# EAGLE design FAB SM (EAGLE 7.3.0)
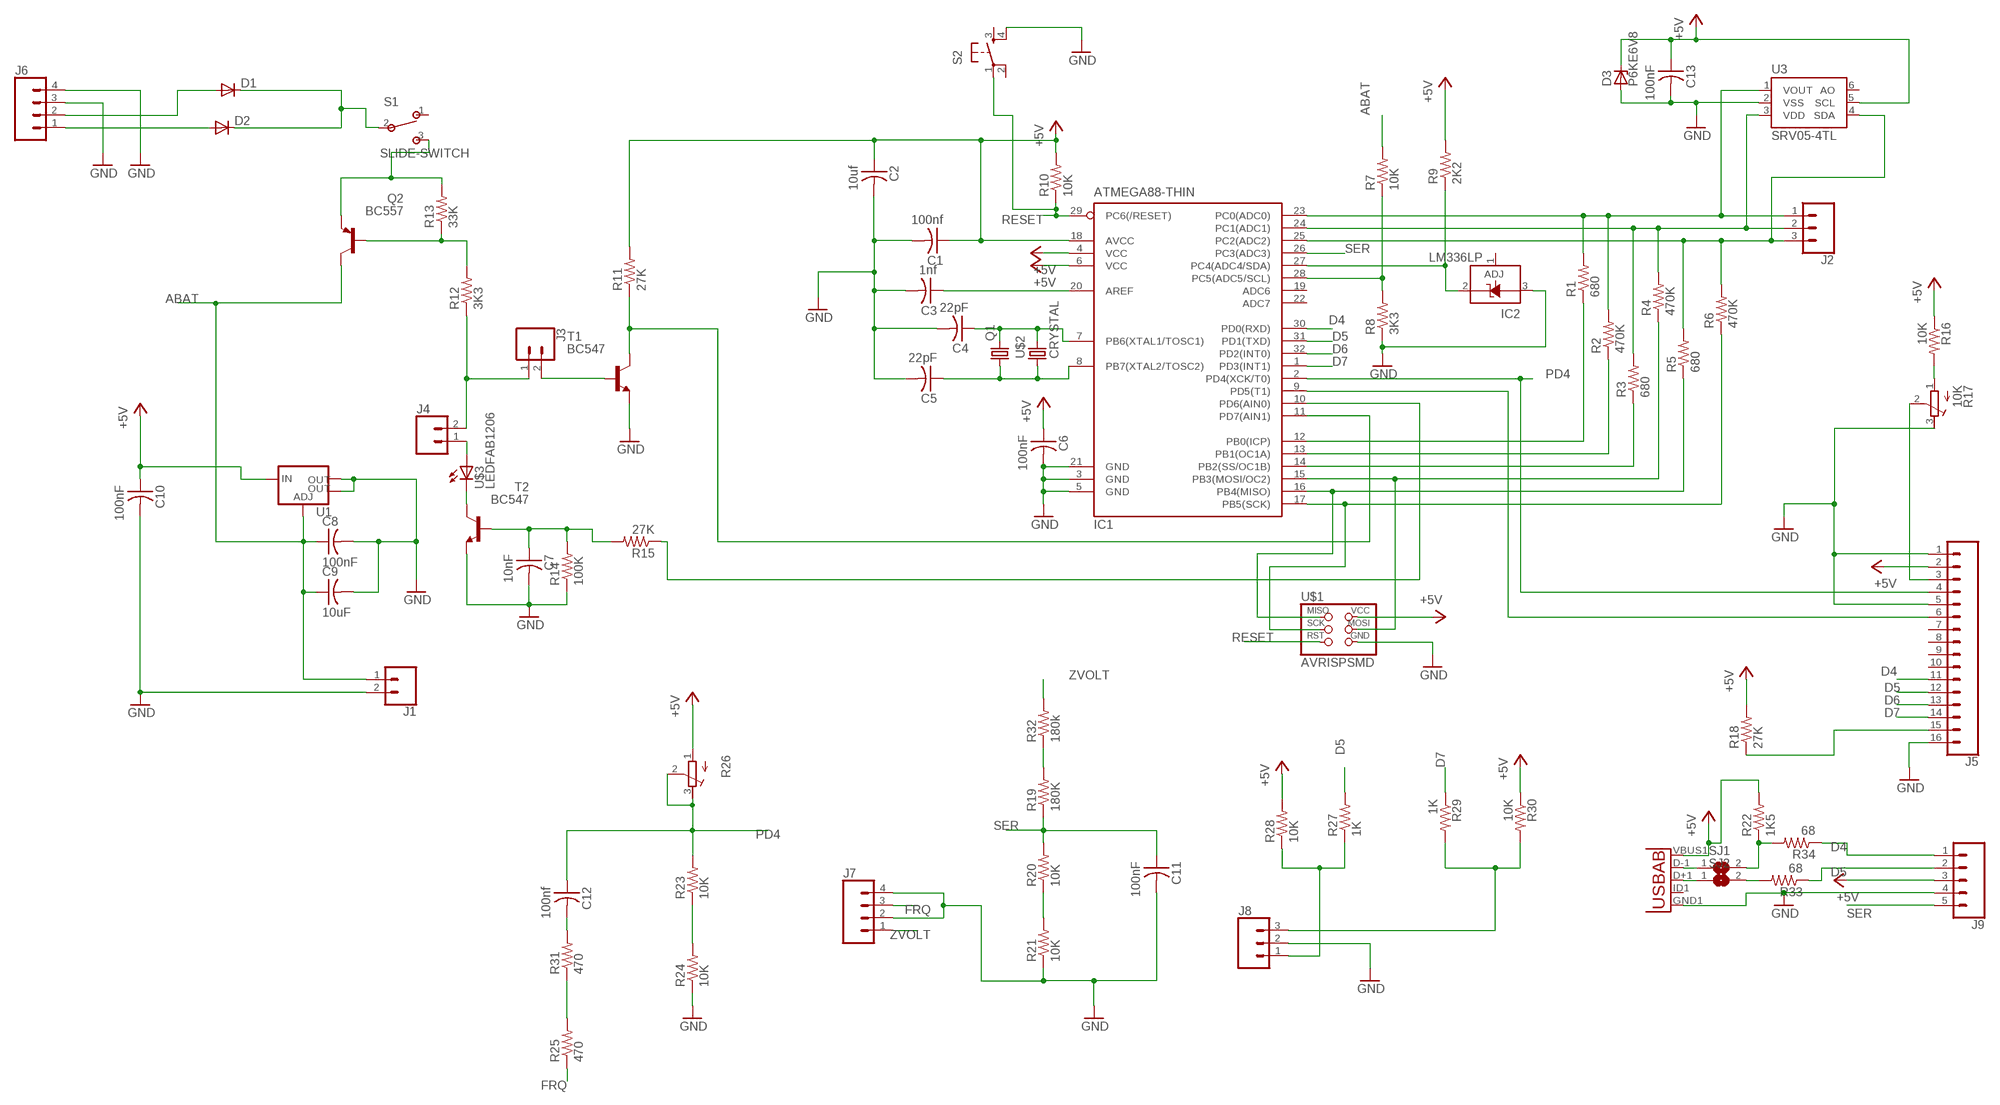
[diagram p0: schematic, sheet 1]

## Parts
C1  100nf  CAP-US1206FAB  [C1206FAB]
C2  10uf  CAP-US1206FAB  [C1206FAB]
C3  1nf  CAP-US1206FAB  [C1206FAB]
C4  22pF  CAP-US1206FAB  [C1206FAB]
C5  22pF  CAP-US1206FAB  [C1206FAB]
C6  100nF  CAP-US1206FAB  [C1206FAB]
C7  10nF  CAP-US1206FAB  [C1206FAB]
C8  100nF  CAP-US1206FAB  [C1206FAB]
C9  10uF  CAP-US1206FAB  [C1206FAB]
C10  100nF  CAP-US1206FAB  [C1206FAB]
C11  100nF  CAP-US1206FAB  [C1206FAB]
C12  100nf  CAP-US1206FAB  [C1206FAB]
C13  100nF  CAP-US1206FAB  [C1206FAB]
D1  DIODESOD123  [SOD123]
D2  DIODESOD123  [SOD123]
D3  P6KE6V8  1N4728  [DO41Z10]
IC1  ATMEGA88-THIN  [TQFP32-08THIN]
IC2  LM336LP  [TO92]
J1  CONN_02PTH3  [1X02_LONGPADS]
J2  CONN_03LOCK_LONGPADS  [1X03_LOCK_LONGPADS]
J3  CONN_02PTH3  [1X02_LONGPADS]
J4  CONN_02PTH3  [1X02_LONGPADS]
J5  CONN_16LONGPADS  [1X16_LONGPADS]
J6  CONN_04LOCK_LONGPADS  [1X04_LOCK_LONGPADS]
J7  CONN_04LOCK_LONGPADS  [1X04_LOCK_LONGPADS]
J8  CONN_03LOCK_LONGPADS  [1X03_LOCK_LONGPADS]
J9  CONN_05LOCK_LONGPADS  [1X05_LOCK_LONGPADS]
Q1  CRYSTALHC49S  [HC49/S]
Q2  BC557  [TO92]
R1  680  RES-US1206FAB  [R1206FAB]
R2  470K  RES-US1206FAB  [R1206FAB]
R3  680  RES-US1206FAB  [R1206FAB]
R4  470K  RES-US1206FAB  [R1206FAB]
R5  680  RES-US1206FAB  [R1206FAB]
R6  470K  RES-US1206FAB  [R1206FAB]
R7  10K  RES-US1206FAB  [R1206FAB]
R8  3K3  RES-US1206FAB  [R1206FAB]
R9  2K2  RES-US1206FAB  [R1206FAB]
R10  10K  RES-US1206FAB  [R1206FAB]
R11  27K  RES-US1206FAB  [R1206FAB]
R12  3K3  RES-US1206FAB  [R1206FAB]
R13  33K  RES-US1206FAB  [R1206FAB]
R14  100K  RES-US1206FAB  [R1206FAB]
R15  27K  RES-US1206FAB  [R1206FAB]
R16  10K  RES-US1206FAB  [R1206FAB]
R17  10K  R-TRIMM64Z  [RTRIM64Z]
R18  27K  RES-US1206FAB  [R1206FAB]
R19  180K  RES-US1206FAB  [R1206FAB]
R20  10K  RES-US1206FAB  [R1206FAB]
R21  10K  RES-US1206FAB  [R1206FAB]
R22  1K5  R-US_0204/7  [0204/7]
R23  10K  RES-US1206FAB  [R1206FAB]
R24  10K  RES-US1206FAB  [R1206FAB]
R25  470  RES-US1206FAB  [R1206FAB]
R26  R-TRIMM64Z  [RTRIM64Z]
R27  1K  RES-US1206FAB  [R1206FAB]
R28  10K  RES-US1206FAB  [R1206FAB]
R29  1K  RES-US1206FAB  [R1206FAB]
R30  10K  RES-US1206FAB  [R1206FAB]
R31  470  R-US_0204/7  [0204/7]
R32  180k  R-US_0204/7  [0204/7]
R33  68  R-US_0204/7  [0204/7]
R34  68  R-US_0204/7  [0204/7]
S1  SLIDE-SWITCH  [AYZ0102AGRLC]
S2  6MM_SWITCH6MM_SWITCH  [6MM_SWITCH]
SJ1  SJ  [SJ]
SJ2  SJ  [SJ]
T1  BC547  [TO92]
T2  BC547  [TO92]
U1  V_REG_LM1117SOT223  [SOT223]
U2  USB""  [USB-MICRO-SMD]
U3  SRV05-4TL  MCP4725SOT-23  [SOT23-6]
U$1  AVRISPSMD  [2X03SMD]
U$2  CRYSTAL  [2-SMD-5X3MM]
U$3  LEDFAB1206  [LED1206FAB]

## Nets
+5V: C1.1 C2.1 C6.1 C10.1 C13.1 D3.C IC1.4(VCC) IC1.6(VCC) IC1.18(AVCC) J5.2 J9.3 R9.2 R10.2 R11.2 R16.1 R18.2 R22.2 R26.1(A) R28.2 R30.1 U1.3(IN) U2.VBUS1(VBUS) U3.5(SCL) U$1.2(VCC)
ABAT: C8.1 C9.1 J1.1 Q2.3(C) R7.2 U1.1(ADJ)
D4: IC1.30(PD0(RXD)) J5.11 J9.1 R34.1
D5: IC1.31(PD1(TXD)) J5.12 J9.2 R27.2 R33.1
D6: IC1.32(PD2(INT0)) J5.13
D7: IC1.1(PD3(INT1)) J5.14 R29.1
FRQ: J7.3 R25.1
GND: C1.2 C2.2 C3.2 C4.2 C5.2 C6.2 C7.2 C8.2 C9.2 C10.2 C11.2 C13.2 D3.A IC1.3(GND) IC1.5(GND) IC1.21(GND) IC2.3(A) J1.2 J5.1 J5.5 J5.16 J6.3 J6.4 J7.2 J7.4 J8.2 J9.4 R8.1 R14.1 R17.3(E) R21.1 R24.1 S2.4(S1) T1.1(E) T2.1(E) U1.2(OUT) U1.4(OUT) U2.GND1(GND) U3.2(VSS) U$1.6(GND)
N$1: IC1.23(PC0(ADC0)) J2.1 R1.2 R2.2 U3.1(VOUT)
N$2: IC1.12(PB0(ICP)) R1.1
N$3: IC1.13(PB1(OC1A)) R2.1
N$4: IC1.14(PB2(SS/OC1B)) R3.1
N$5: IC1.15(PB3(MOSI/OC2)) R4.1 U$1.4(MOSI)
N$6: IC1.16(PB4(MISO)) R5.1 U$1.1(MISO)
N$7: IC1.17(PB5(SCK)) R6.1 U$1.3(SCK)
N$8: IC1.24(PC1(ADC1)) J2.2 R3.2 R4.2 U3.3(VDD)
N$9: IC1.25(PC2(ADC2)) J2.3 R5.2 R6.2 U3.4(SDA)
N$10: IC1.28(PC5(ADC5/SCL)) R7.1 R8.2
N$11: IC1.27(PC4(ADC4/SDA)) IC2.2(C) R9.1
N$12: C3.1 IC1.20(AREF)
N$13: IC1.11(PD7(AIN1)) R11.1 T1.3(C)
N$14: C4.1 IC1.7(PB6(XTAL1/TOSC1)) Q1.2 U$2.P$2
N$15: C5.1 IC1.8(PB7(XTAL2/TOSC2)) Q1.1 U$2.P$1
N$17: J3.2 T1.2(B)
N$18: J3.1 J4.2 R12.1
N$19: Q2.2(B) R12.2 R13.1
N$20: D1.CATHODE(C) D2.CATHODE(C) S1.2
N$21: J4.1 U$3.1(A)
N$22: T2.3(C) U$3.2(C)
N$24: C7.1 R14.2 R15.2 T2.2(B)
N$25: R16.2 R17.1(A)
N$26: IC1.10(PD6(AIN0)) R15.1
N$27: R20.1 R21.2
N$28: J5.3 R17.2(S)
N$29: J8.1 R27.1 R28.1
N$30: J5.15 R18.1
N$31: IC1.9(PD5(T1)) J5.6
N$32: D1.ANODE(A) J6.2
N$33: D2.ANODE(A) J6.1
N$34: R19.2 R32.1
N$35: R23.1 R24.2
N$36: Q2.1(E) R13.2 S1.3
N$37: J8.3 R29.2 R30.2
N$38: R25.2 R31.1
N$39: C12.2 R31.2
N$40: SJ1.1 U2.D-1(D-)
N$42: SJ2.1 U2.D+1(D+)
N$43: R33.2 SJ2.2
N$45: R22.1 R34.2 SJ1.2
PD4: C12.1 IC1.2(PD4(XCK/T0)) J5.4 R23.2 R26.2(S) R26.3(E)
RESET: IC1.29(PC6(/RESET)) R10.1 S2.1(P) U$1.5(RST)
SER: C11.1 IC1.26(PC3(ADC3)) J9.5 R19.1 R20.2
ZVOLT: J7.1 R32.2
Unconnected: IC1.19(ADC6) IC1.22(ADC7) IC2.1(ADJ) J5.7 J5.8 J5.9 J5.10 S1.1 S2.2(P1) S2.3(S) U2.ID1(USBID) U3.6(AO)

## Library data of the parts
C1-C13 = fab:CAP-US
D1 D2 = fab:DIODE: DIODE
D3 = diode:1N4728: Z DIODE
IC1 = fab:ATMEGA88-THIN
IC2 = linear:LM336: 2.5-V INTEGRATED REFERENCE CIRCUITS LM236 Source: http://focus.ti.com/lit/ds/symlink/lm336-2.5.pdf
J1 J3 J4 = SparkFun-Connectors:CONN_02: Multi connection point. Often used as Generic Header-pin footprint for 0.1 inch spaced/style header connections
J2 J8 = SparkFun-Connectors:CONN_03: Multi connection point. Often used as Generic Header-pin footprint for 0.1 inch spaced/style header connections On any of the 0.1 inch spaced packages, you can populate with these: Break Away Headers - Straight (PRT-00116) Break Away Male Headers - Right Angle (PRT-00553) Female Headers (PRT-00115)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
J5 = SparkFun-Connectors:CONN_16: Multi connection point. Often used as Generic Header-pin footprint for 0.1 inch spaced/style header connections On any of the 0.1 inch spaced packages, you can populate with these: Break Away Headers - Straight (PRT-00116) Break Away Male Headers - Right Angle (PRT-00553) Female Headers (PRT-00115)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
J6 J7 = SparkFun-Connectors:CONN_04: Multi connection point. Often used as Generic Header-pin footprint for 0.1 inch spaced/style header connections On any of the 0.1 inch spaced packages, you can populate with these: Break Away Headers - Straight (PRT-00116) Break Away Male Headers - Right Angle (PRT-00553) Female Headers (PRT-00115)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; PROD_ID: CONN-09696
J9 = SparkFun-Connectors:CONN_05: Multi connection point. Often used as Generic Header-pin footprint for 0.1 inch spaced/style header connections On any of the 0.1 inch spaced packages, you can populate with these: Break Away Headers - Straight (PRT-00116) Break Away Male Headers - Right Angle (PRT-00553) Female Headers (PRT-00115)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
Q1 = crystal:CRYSTAL: CRYSTAL; OC_FARNELL: 1667008; OC_NEWARK: unknown
Q2 = transistor-pnp:BC557: PNP Transistor
R1-R16 R18-R21 R23-R25 R27-R30 = fab:RES-US: Resistor (US Symbol)
R17 R26 = resistor:R-TRIMM: Trimm resistor
R22 R31-R34 = resistor:R-US_: RESISTOR, American symbol
S1 = fab:SLIDE-SWITCH: SMD slide-switch AYZ0102AGRLC as found in the fablab inventory. Includes the mounting holes. Made by Zaerc.
S2 = fab:6MM_SWITCH: OMRON SWITCH
SJ1 SJ2 = jumper:SJ: SMD solder JUMPER
T1 T2 = transistor:BC547: NPN TRANSISTOR
U1 = fab:V_REG_LM1117: Voltage Regulator LM1117 Standard adjustable voltage regulator but in SMD form. Spark Fun Electronics SKU : COM-00595; PROD_ID: VREG-08170
U2 = MicroUSB:USB: This is a USB AB connector that is compatible with USB OTG. i.e. this connector can serve as a host or device
U3 = SparkFun-IC-Conversion:MCP4725: MCP4725 DAC Microchip 12-bit I2C DAC, SOT23-6 Datasheet SparkFun Products SparkFun I2C DAC Breakout - MCP4725 (BOB-12918); PROD_ID: IC-08886; VALUE: MCP4725
U$1 = fab:AVRISP
U$2 = fab:CRYSTAL
U$3 = fab:LED: LED

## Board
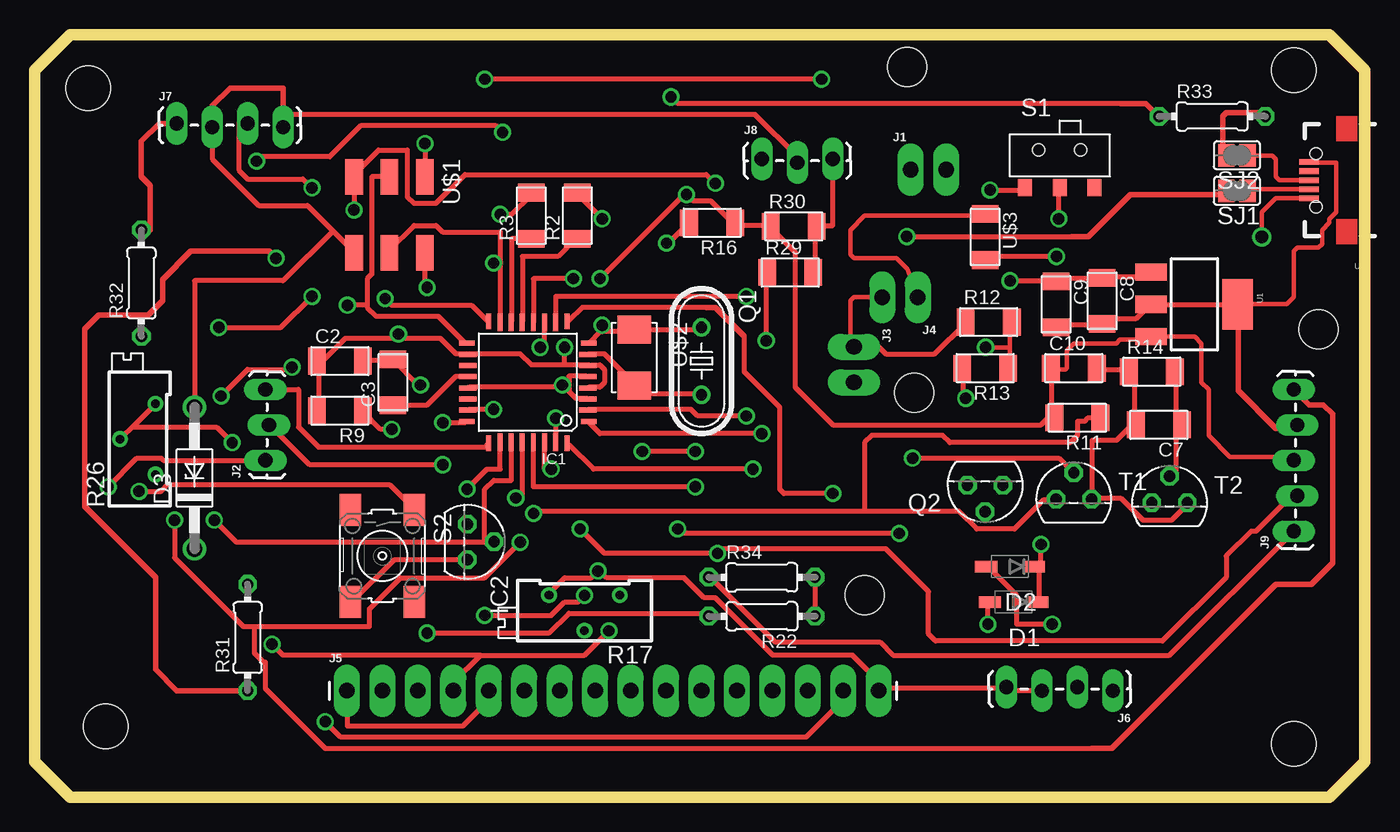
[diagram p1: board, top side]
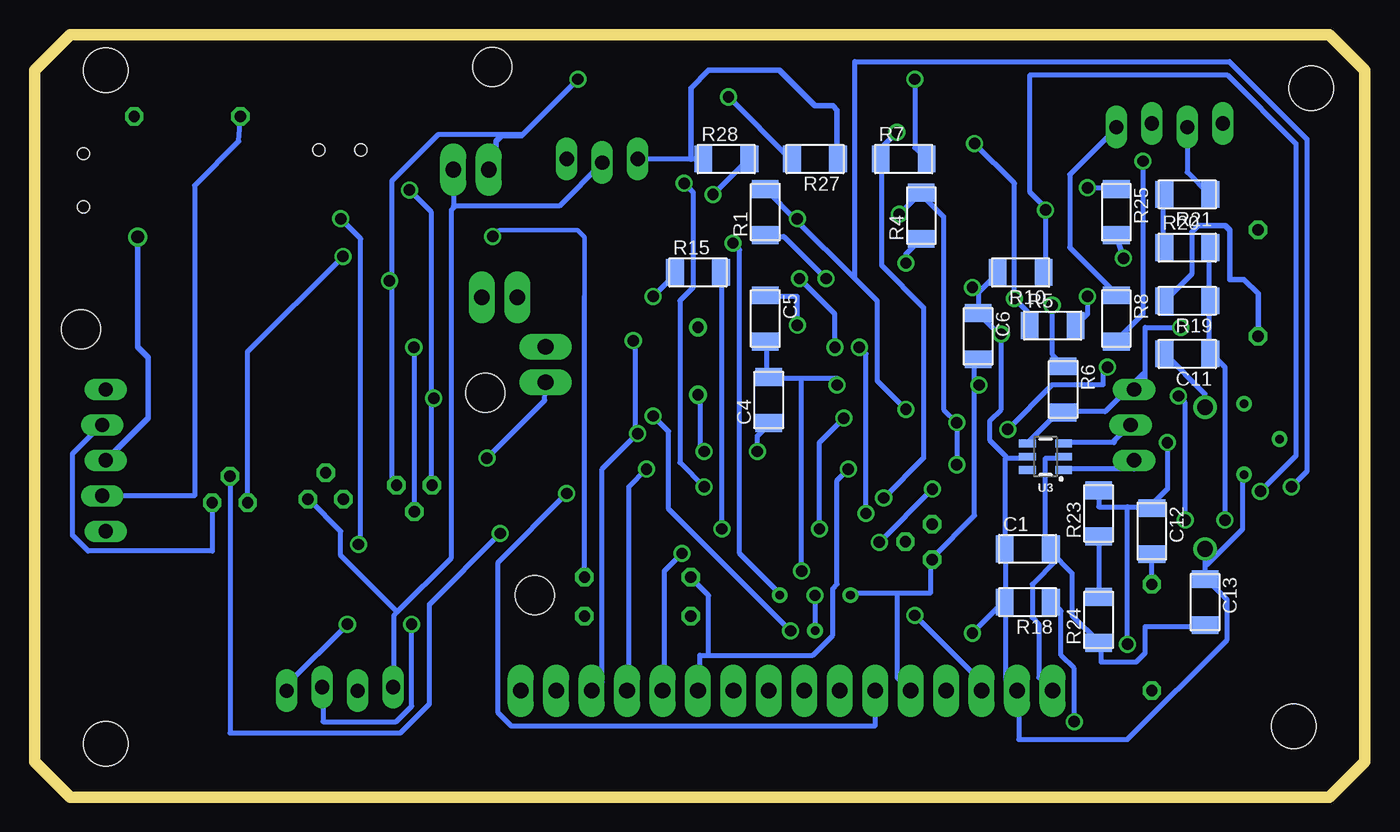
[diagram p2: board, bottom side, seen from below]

Size 95.25 x 54.61 mm. Coordinates in mm from the lower left corner, seen from the top.
Outline: 0,2.54 0,52.07 2.54,54.61 92.71,54.61 95.25,52.07 95.25,2.54 92.71,0 2.54,0 0,2.54
Copper layers (1*16): Top 0.035mm / dielectric 1.5mm / Bottom 0.035mm
Design rules "default *": minimum track width 14mil, minimum drill 32mil, track to track 14mil, track to pad 15mil, pad to pad 16mil, via to via 18mil, smd to smd 14mil, copper to edge 40mil, drill to drill 18mil, minimum pad ring 10mil, minimum via ring 8mil, stop-mask expansion 4mil, vias tented up to drill 0mil, thermal gap 10mil
Holes 3.2 mm at 5.08,5.08 90.17,3.81 90.17,52.07 3.81,50.8
Holes 2.8 mm at 59.44,14.48 62.99,28.96 62.48,52.32 91.95,33.53

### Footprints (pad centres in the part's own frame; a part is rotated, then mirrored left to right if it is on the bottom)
C1206FAB = smd 1.27 x 1.905: 1 -1.651,0; 2 1.651,0
SOD123 = smd 1.6 x 0.8: ANODE 1.7,0; CATHODE -1.7,0
DO41Z10 = drill 1.118: A 5.08,0; C -5.08,0
TQFP32-08THIN = smd 1.118 x 0.356: 1 -4.369,2.8; 8 -4.369,-2.8; 17 4.369,-2.8; 24 4.369,2.8 | smd 1.27 x 0.356: 2 -4.293,2; 3 -4.293,1.2; 4 -4.293,0.4; 5 -4.293,-0.4; 6 -4.293,-1.2; 7 -4.293,-2; 18 4.293,-2; 19 4.293,-1.2; 20 4.293,-0.4; 21 4.293,0.4; 22 4.293,1.2; 23 4.293,2 | smd 0.356 x 1.118: 9 -2.8,-4.369; 16 2.8,-4.369; 25 2.8,4.369; 32 -2.8,4.369 | smd 0.356 x 1.27: 10 -2,-4.293; 14 1.2,-4.293; 15 2,-4.293; 26 2,4.293; 27 1.2,4.293; 31 -2,4.293 | smd 0.35 x 1.27: 11 -1.2,-4.293; 12 -0.4,-4.293; 13 0.4,-4.293; 28 0.4,4.293; 29 -0.4,4.293; 30 -1.2,4.293
TO92 = drill 0.813 octagon: 1 -1.27,0; 2 0,1.905; 3 1.27,0
1X02_LONGPADS = drill 1.118 pad 1.88 long: 1 0,0; 2 2.54,0
1X03_LOCK_LONGPADS = drill 1.016 long: 1 0,0; 2 2.54,-0.254; 3 5.08,0
1X16_LONGPADS = drill 1.118 pad 1.88 long: 1 0,0; 2 2.54,0; 3 5.08,0; 4 7.62,0; 5 10.16,0; 6 12.7,0; 7 15.24,0; 8 17.78,0; 9 20.32,0; 10 22.86,0; 11 25.4,0; 12 27.94,0; 13 30.48,0; 14 33.02,0; 15 35.56,0; 16 38.1,0
1X04_LOCK_LONGPADS = drill 1.016 long: 1 0,0; 2 2.54,-0.254; 3 5.08,0; 4 7.62,-0.254
1X05_LOCK_LONGPADS = drill 1.016 long: 1 0,0; 2 2.54,-0.254; 3 5.08,0; 4 7.62,-0.254; 5 10.16,0
HC49/S = drill 0.813: 1 -2.413,0; 2 2.413,0
TO92' = drill 0.813 octagon: 1 1.27,0; 2 0,1.905; 3 -1.27,0
R1206FAB = smd 1.27 x 1.905: 1 -1.651,0; 2 1.651,0
RTRIM64Z = drill 0.61: 1 0,-2.54; 2 -2.54,0; 3 0,2.54
0204/7 = drill 0.813 octagon: 1 -3.81,0; 2 3.81,0
AYZ0102AGRLC = smd 1 x 1.2: 1 2.5,-2.3; 2 0,-2.3; 3 -2.5,-2.3 | hole 0.85: -1.5,0.4; 1.5,0.4
6MM_SWITCH = smd 2.286 x 1.524: 1 -3.302,2.286; 2 3.302,2.286; 3 -3.302,-2.286; 4 3.302,-2.286
SJ = smd 1.168 x 1.6: 1 -0.762,0; 2 0.762,0
SOT223 = smd 1.219 x 2.235: 1 -2.311,-3.099; 2 0,-3.099; 3 2.311,-3.099 | smd 3.6 x 2.2: 4 0,3.099
USB-MICRO-SMD = smd 1.4 x 0.4: D+1 2.7,0; D-1 2.7,0.65; GND1 2.7,-1.3; ID1 2.7,-0.65; VBUS1 2.7,1.3 | hole 0.85: 2.2,1.9; 2.2,-1.9
SOT23-6 = smd 0.55 x 1.2: 1 0.95,1.3; 2 0,1.3; 3 -0.95,1.3; 4 -0.95,-1.3; 5 0,-1.3; 6 0.95,-1.3
2X03SMD = smd 2.54 x 1.27: 1 -2.54,2.54; 2 2.92,2.54; 3 -2.54,0; 4 2.92,0; 5 -2.54,-2.54; 6 2.92,-2.54
2-SMD-5X3MM = smd 2 x 2.4: P$1 -2,0; P$2 2,0
LED1206FAB = smd 1.27 x 1.905: 1 -1.651,0; 2 1.651,0

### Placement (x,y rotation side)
C1  24.13,17.78 0 bottom
C2  21.84,31.24 0 top
C3  25.65,29.72 90 top
C4  42.67,28.45 90 bottom
C5  42.93,34.29 270 bottom
C6  27.69,33.02 270 bottom
C7  80.52,26.67 180 top
C8  76.45,35.56 270 top
C9  73.15,35.31 270 top
C10  74.42,30.73 0 top
C11  12.7,31.75 180 bottom
C12  15.24,19.05 270 bottom
C13  11.43,13.97 270 bottom
D1  70.1,13.97 180 top
D2  69.85,16.51 180 top
D3  11.43,22.86 90 top
IC1  35.31,29.72 180 top
IC2  30.99,18.29 270 top
J1  62.74,44.96 0 top
J2  16.51,24.13 90 top
J3  58.67,32.26 270 top
J4  63.25,35.81 180 top
J5  22.35,7.62 0 top
J6  77.22,7.62 180 top
J7  10.16,48.26 0 top
J8  52.07,45.72 0 top
J9  90.17,19.05 90 top
Q1  47.75,31.24 270 top
Q2  BC557  [TO92']  68.07,22.35 180 top
R1  42.93,41.91 90 bottom
R2  38.86,41.66 90 top
R3  35.56,41.66 90 top
R4  31.75,41.66 90 bottom
R5  22.35,33.78 0 bottom
R6  21.59,29.21 270 bottom
R7  33.02,45.72 0 bottom
R8  17.78,34.29 270 bottom
R9  21.84,27.69 180 top
R10  24.64,37.59 180 bottom
R11  74.68,27.18 180 top
R12  68.33,34.04 0 top
R13  68.07,30.73 180 top
R14  80.01,30.48 0 top
R15  47.75,37.59 0 bottom
R16  48.51,41.15 180 top
R17  39.37,14.48 90 top
R18  24.13,13.97 180 bottom
R19  12.7,35.56 180 bottom
R20  12.7,39.37 0 bottom
R21  12.7,43.18 180 bottom
R22  52.07,12.95 180 top
R23  19.05,20.32 90 bottom
R24  19.05,12.7 90 bottom
R25  17.78,41.91 270 bottom
R26  8.64,25.65 0 top
R27  39.37,45.72 180 bottom
R28  45.72,45.72 0 bottom
R29  54.1,37.59 0 top
R30  54.36,40.89 0 top
R31  15.24,11.43 90 top
R32  7.62,36.83 90 top
R33  84.33,48.77 0 top
R34  52.07,15.75 0 top
S1  73.41,45.97 0 top
S2  24.89,17.27 270 top
SJ1  86.11,43.43 180 top
SJ2  86.11,45.97 180 top
T1  BC547  [TO92']  74.42,21.34 0 top
T2  BC547  [TO92']  81.28,21.08 0 top
U1  83.06,35.31 270 top
U2  93.98,44.2 180 top
U3  22.86,24.38 270 bottom
U$1  25.4,41.91 270 top
U$2  42.93,31.5 270 top
U$3  68.07,40.13 270 top

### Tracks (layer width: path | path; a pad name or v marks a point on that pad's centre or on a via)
+5V  (via drill 0.81, 0.9)
  Top 0.305: v87.88,40.13 87.88,41.91 88.9,42.93 91.25,42.93 U2.VBUS1 | 72.87,30.64 73.82,30.64 73.91,30.73 73.91,32 74.42,32.51 77.47,32.51 77.72,32.77 79.73,32.77 U1.3 83.08,32.99 83.57,32.51 83.57,29.72 84.07,29.21 84.07,25.91 85.6,24.38 89.92,24.38 J9.3
  Top 0.356: C10.1 72.87,30.64 72.87,27.3 73.02,27.3 R11.2 72.71,27.3 72.07,26.67 57.15,26.67 54.45,29.37 54.45,39.05 52.71,40.8 R30.1 52.71,40.96 50.32,40.96 50.16,41.12 R16.1 50.01,41.12 48.42,42.7 47.15,42.7 v46.67,43.18 46.51,43.18 v40.48,37.15 | R9.2 20.32,27.78 20.32,31.11 C2.1 20.48,31.11 22.22,32.86 26.04,32.86 | IC1.4 39.69,29.37 40.48,29.37 40.8,29.69 40.8,30.64 40.48,30.96 39.69,30.96 IC1.6 39.53,30.96 37.94,30.96 | 37.94,30.96 35.56,30.96 34.77,31.75 31.11,31.75 IC1.18 30.96,31.75 30.16,31.75 29.05,32.86 26.04,32.86 | U$1.2 27.94,36.51 v28.1,36.51 | v28.1,11.75 36.83,11.75 38.26,13.18 48.1,13.18 48.26,13.02 R22.2 | v26.04,33.18 26.04,32.86 | 37.94,30.96 v37.94,32.23
  Bottom 0.356: v46.67,43.18 44.13,45.72 R28.2 | D3.C 11.43,16.67 | 11.43,16.67 C13.1 11.27,15.56 9.84,14.13 9.84,11.27 16.99,4.13 24.76,4.13 24.76,7.62 J5.2 24.92,7.62 25.72,8.41 25.72,13.81 R18.2 | R26.1 8.73,23.02 8.73,19.21 11.27,16.67 11.43,16.67 | 27.62,36.2 26.35,37.47 R10.2 | 27.62,36.2 27.62,34.77 C6.1 26.11,33.1 | v28.1,36.51 27.78,36.2 27.62,36.2 | 25.72,24.29 24.29,24.29 U3.5 | 25.72,24.29 25.72,17.78 C1.1 25.72,17.62 25.72,13.97 R18.2 | v28.1,11.75 25.88,13.97 R18.2 | 26.11,33.1 26.04,33.02 26.04,27.78 26.83,26.99 26.83,25.56 25.72,24.45 25.72,24.29 | v26.04,33.18 26.11,33.1 | v40.48,37.15 37.94,34.61 v37.94,32.23
  Bottom 0.406: v87.88,40.13 87.88,32.26 87.12,31.5 87.12,27.18 J9.3
ABAT  (via drill 0.81)
  Top 0.356: U1.1 79.85,37.47 79.69,37.31 76.52,37.31 C8.1 76.36,37.15 73.34,37.15 C9.1 73.02,36.99 v69.85,36.99 | v56.36,51.44 v32.23,51.44
  Bottom 0.356: v32.23,51.44 32.23,46.51 31.43,45.72 R7.2 | v56.36,51.44 60.4,47.39 60.48,47.47 66.36,47.47 69.69,44.13 69.69,36.99 | 62.71,45.09 J1.1 | Q2.3 69.69,22.7 69.69,36.99 | v69.85,36.99 69.69,36.99
  Bottom 0.406: 60.4,47.39 61.83,47.39 62.23,46.99 62.23,45.47 J1.1
D4  (via drill 0.81)
  Top 0.356: v36.99,23.5 36.51,23.5 36.51,25.4 IC1.30 | R34.1 48.26,15.72 48.42,15.72 53.02,11.11 60.52,11.11 61.47,10.16 81.28,10.16 J9.1
  Bottom 0.356: v36.99,23.5 37.78,22.7 37.78,15.24 38.1,14.92 38.1,11.59 39.53,10.16 46.99,10.16 | 46.99,10.16 47.62,10.16 47.62,7.62 J5.11 | 46.99,10.16 46.99,14.45 48.26,15.72 R34.1
D5  (via drill 0.81)
  Top 0.356: v37.31,27.15 37.31,25.56 IC1.31 | v39.05,19.21 40.8,17.46 v48.9,17.46 | v45.56,50.16 46.04,49.69 77.79,49.69 | 49.21,17.62 49.05,17.46 v48.9,17.46 | J9.2 90.01,21.59 87.47,19.05 87.12,19.05 85.34,17.27 85.34,15.75 80.77,11.18 64.52,11.18 64.01,11.68 64.01,14.73 60.96,17.78 49.21,17.78 v48.9,17.46
  Top 0.406: 77.79,49.69 79.6,49.69 R33.1
  Bottom 0.356: v37.31,27.15 39.05,25.4 v39.05,19.21 | v48.9,17.46 50.16,16.19 50.16,7.62 J5.12 | v45.56,50.16 41.12,45.72 R27.2 | J9.2 83.82,21.59 83.82,43.81 80.64,46.99 R33.1
D6  (via drill 0.81)
  Top 0.356: v51.44,23.5 40.01,23.5 38.26,25.24 IC1.32
  Bottom 0.356: v51.44,23.5 52.71,22.23 52.71,7.62 J5.13
D7  (via drill 0.81)
  Top 0.356: v52.07,26.04 40.48,26.04 39.69,26.83 IC1.1 | v52.39,32.7 52.39,37.47 R29.1
  Bottom 0.356: J5.14 55.25,7.62 54.61,8.26 54.61,23.5 v52.07,26.04 52.23,26.04 52.23,32.54 v52.39,32.7
FRQ  (via drill 0.81)
  Top 0.356: v19.84,43.66 19.21,44.29 15.24,44.29 14.61,44.93 14.61,48.26 J7.3
  Bottom 0.356: v19.84,43.66 17.78,43.66 R25.1
GND  (via drill 0.81)
  Top 0.305: U1.4 89.66,35.31 90.17,35.81 90.17,39.12 90.42,39.37 91.95,39.37 92.2,39.62 92.2,40.64 92.71,41.15 92.71,41.4 93.22,41.91 93.22,45.47 91.31,45.47 U2.GND1
  Top 0.356: 38.26,29.37 38.26,30.16 39.53,30.16 IC1.5 | 38.26,29.37 38.26,29.05 38.73,28.57 39.53,28.57 IC1.3 | 38.26,29.37 37.78,29.37 | 37.78,29.37 31.11,29.37 IC1.21 | v37.78,29.53 37.78,29.37 | C2.2 23.49,31.27 25.56,31.27 C3.2 25.72,31.27 27.46,29.53 v27.62,29.53 | S2.4 22.7,13.97 25.72,16.99 30.96,16.99 IC2.3 | R17.3 36.83,14.61 37.94,15.72 39.85,15.72 v40.32,16.19 40.48,16.19 40.96,15.72 46.51,15.72 47.94,14.29 48.74,14.29 52.86,10.16 58.58,10.16 60.8,7.94 J5.16 60.48,7.62 60.64,7.78 69.53,7.78 J6.4 69.85,7.62 J6.3 | J5.1 22.38,7.62 22.38,5.08 30.64,5.08 32.39,6.83 32.39,7.62 J5.5 | 21.35,40.56 19.53,42.39 16.03,42.39 12.7,45.72 J7.2 12.7,48.42 | 21.35,40.56 22.86,39.05 U$1.6 | D3.A 11.43,36.99 17.78,36.99 21.35,40.56 | C9.2 73.18,33.66 73.34,33.81 76.36,33.81 C8.2 76.83,34.29 78.9,34.29 79.85,35.24 U1.2 80.01,35.24 86.04,35.24 U1.4 86.2,35.24 | C10.2 76.2,30.64 78.1,30.64 78.26,30.48 R14.1 78.42,30.32 78.74,30.32 78.74,26.67 C7.2 78.58,26.67 77.47,25.56 75.72,25.56 75.72,21.43 T1.1 75.88,21.43 77.79,21.43 79.38,19.84 81.44,19.84 82.55,20.95 T2.1 | J8.2 54.61,45.88 51.59,48.9 17.94,48.9 J7.4
  Top 0.406: J7.4 17.78,50.8 13.97,50.8 12.7,49.53 J7.2 | 86.2,35.24 86.2,29.11 88.9,26.42 90.17,26.42 J9.4
  Bottom 0.356: U3.2 21.59,24.29 22.86,24.29 22.86,18.1 22.54,17.78 C1.2 | C1.2 22.54,17.62 20.95,16.03 20.95,13.02 19.05,11.11 R24.1 18.89,11.11 18.89,9.68 16.35,9.68 15.72,10.32 15.72,12.22 11.43,12.22 C13.2 | J5.1 22.38,7.62 23.34,8.57 23.34,12.38 23.81,12.86 23.81,15.24 22.07,16.99 C1.2 | C5.2 42.86,32.54 42.86,30.32 42.7,30.16 C4.2 42.55,30 40.32,30 | 40.32,30 37.78,30 v37.78,29.53 | C6.2 27.94,31.11 27.94,29.53 | 27.94,29.53 27.94,20.16 30.96,17.14 IC2.3 31.11,16.99 31.11,14.61 33.5,14.61 | 33.5,14.61 36.83,14.61 R17.3 | v27.62,29.53 27.94,29.53 | 33.5,14.61 33.5,8.57 32.54,7.62 J5.5 | v40.32,16.19 40.32,30 | R8.1 17.78,36.04 21.11,39.37 21.11,44.61 17.78,47.94 J7.4 | D3.A 11.43,28.89 14.29,31.75 C11.2 | J7.2 12.7,44.77 11.11,43.18 R21.1 | 65.25,42.39 57.63,42.39 54.61,45.4 J8.2 | 65.25,42.39 65.25,44.93 J1.2 | 69.29,13.26 69.53,13.02 69.53,7.94 J6.4 | 69.29,13.26 65.41,17.14 65.41,42.07 65.25,42.23 65.25,42.39 | 69.29,13.26 73.34,17.3 73.34,19.05 75.56,21.27 T1.1 | T2.1 82.55,17.62 91.44,17.62 92.55,18.73 92.55,24.61 90.49,26.67 J9.4
N$1  (via drill 0.81)
  Top 0.356: v32.86,27.78 31.11,27.78 IC1.23 | v40.64,41.43 38.89,43.18 R2.2 | J2.1 9.21,24.13 9.05,24.29 7.3,24.29 v5.24,22.23
  Bottom 0.356: J2.1 16.51,23.5 21.43,23.5 U3.1 | v32.86,27.78 34.93,29.84 34.93,35.56 36.59,37.23 | R1.2 40.72,41.35 | 40.72,41.35 36.59,37.23 | v40.64,41.43 40.72,41.35 | v5.24,22.23 4.13,23.34 4.13,47.15 9.68,52.7 36.51,52.7 36.51,37.31 36.59,37.23
N$2  (via drill 0.81)
  Top 0.356: v38.58,37.15 35.72,37.15 35.72,34.13 IC1.12
  Bottom 0.356: v38.58,37.15 41.59,40.16 42.86,40.16 R1.1
N$3
  Top 0.356: IC1.13 34.93,34.13 34.93,38.73 37.47,38.73 38.73,40.01 R2.1
N$4
  Top 0.356: R3.1 34.13,40.01 34.13,34.13 IC1.14
N$5  (via drill 0.81)
  Top 0.356: 33.34,38.26 33.34,40.48 29.21,40.48 28.73,40.96 27.15,40.96 25.4,39.21 U$1.4 | 33.34,38.26 33.34,34.13 IC1.15 | 33.34,38.26 v32.86,38.26
  Bottom 0.356: R4.1 32.86,38.89 v32.86,38.26
N$6  (via drill 0.81)
  Top 0.356: v25.08,35.72 25.56,35.24 31.27,35.24 32.39,34.13 IC1.16 | v27.94,46.83 U$1.1
  Bottom 0.356: R5.1 24.13,33.81 24.13,34.77 v25.08,35.72 25.08,43.97 v27.94,46.83
N$7  (via drill 0.81)
  Top 0.356: 23.81,35.24 23.81,37.15 24.13,37.47 24.13,44.45 U$1.3 | 23.81,35.24 23.81,35.08 24.45,34.45 28.89,34.45 30.8,32.54 IC1.17 | 23.81,35.24 v22.38,35.24
  Bottom 0.356: v22.38,35.24 22.38,31.75 21.59,30.96 R6.1
N$8  (via drill 0.81)
  Top 0.356: v29.21,26.83 30.8,26.83 IC1.24 | v33.34,41.75 34.13,41.75 35.56,43.18 R3.2 | v29.21,23.81 19.68,23.81 16.83,26.67 J2.2
  Bottom 0.356: U3.3 21.43,25.4 17.94,25.4 17.94,25.56 16.83,26.67 J2.2 | v33.34,41.75 31.91,43.18 R4.2 31.75,43.18 30.16,41.59 30.16,27.78 v29.21,26.83 v29.21,23.81
N$9  (via drill 0.81)
  Top 0.356: J2.3 18.89,29.21 18.89,26.51 20.32,25.08 32.23,25.08 32.39,25.24 IC1.25 | v19.84,35.88 17.62,33.66 v13.18,33.66
  Bottom 0.356: U3.4 24.13,25.4 22.07,27.46 21.59,27.46 R6.2 21.43,27.62 18.57,27.62 15.88,30.32 15.72,30.32 | v19.84,35.88 19.84,34.61 20.64,33.81 R5.2 | v13.18,33.66 15.72,33.66 15.72,30.32 | 15.72,30.32 15.72,30 J2.3
N$10  (via drill 0.81)
  Top 0.356: v34.45,21.43 34.93,21.43 34.93,25.4 IC1.28 | v15.88,45.56 16.19,45.88 21.11,45.88 23.34,48.1 33.02,48.1 v33.5,47.62
  Bottom 0.356: v34.45,21.43 31.59,24.29 31.59,35.08 34.61,38.1 34.61,45.72 R7.1 34.61,45.88 34.61,46.51 v33.5,47.62 | v15.88,45.56 15.88,34.61 17.78,32.7 R8.2
N$11  (via drill 0.81)
  Top 0.356: 32.23,18.41 32.23,22.07 32.86,22.7 34.13,22.7 34.13,25.4 IC1.27 | 32.23,18.41 32.86,18.41 IC2.2 | v25.56,26.35 24.76,26.35 23.49,27.62 R9.1 | v18.41,30.8 18.26,30.64 15.24,30.64 v13.33,28.73 | v12.86,19.84 14.45,18.26 32.23,18.26 32.23,18.41
  Bottom 0.356: v25.56,26.35 22.38,29.53 18.73,29.53 18.73,30.48 v18.41,30.8 | v13.33,28.73 12.86,28.26 v12.86,19.84
N$12
  Top 0.356: IC1.20 30.96,30.16 30.16,30.16 28.1,28.1 25.72,28.1 C3.1
N$13  (via drill 0.81)
  Top 0.356: v36.2,32.23 36.51,32.23 36.51,33.97 IC1.11 | v35.72,20.32 35.88,20.48 59.44,20.48 | 59.44,20.48 66.2,20.48 67.47,19.21 70.17,19.21 72.23,21.27 73.02,21.27 T1.3 | R11.1 76.2,27.15 75.41,27.15 75.18,26.92 74.68,26.92 74.68,25.91 74.17,25.4 65.53,25.4 65.02,25.91 59.94,25.91 59.44,25.4 59.44,20.48
  Bottom 0.356: v36.2,32.23 35.72,31.75 v35.72,20.32
N$14  (via drill 0.81)
  Top 0.356: IC1.7 39.69,31.75 40.8,31.75 43.02,29.53 U$2.P$2 43.18,29.53 43.82,28.89 47.62,28.89 Q1.2 | v47.31,24.77 v43.5,24.77
  Bottom 0.356: v43.5,24.77 43.5,25.88 42.7,26.67 C4.1 | v47.31,24.77 47.62,25.08 47.62,28.73 Q1.2
N$15  (via drill 0.81)
  Top 0.356: 40.64,33.34 42.86,33.34 U$2.P$1 43.02,33.5 47.47,33.5 47.62,33.66 Q1.1 | 40.64,33.34 40.48,33.34 39.69,32.54 IC1.8 | 40.64,33.34 v40.64,33.81
  Bottom 0.356: v40.64,33.81 40.64,35.88 42.86,35.88 C5.1
N$17  (via drill 0.81)
  Top 0.356: v62.87,24.29 73.34,24.29 74.3,23.34 T1.2
  Bottom 0.356: v62.87,24.29 58.74,28.42 J3.2
N$18
  Top 0.305: J3.1 58.42,32.51 58.42,35.56 58.67,35.81 J4.2
  Top 0.356: R12.1 66.67,33.97 64.45,31.75 60.96,31.75 60.45,32.26 J3.1
N$19  (via drill 0.81)
  Top 0.305: v68.1,32.23 69.82,32.23 69.85,32.26 | 69.85,32.26 69.85,30.86 R13.1 | 69.85,32.26 69.85,33.91 R12.2
  Top 0.356: 69.85,30.8 R13.1 | 69.85,33.97 R12.2
  Bottom 0.356: v68.1,32.23 68.1,20.48 Q2.2
N$20  (via drill 0.81)
  Top 0.356: v73.34,41.43 73.34,43.66 S1.2 | v72.07,18.1 72.07,16.51 D2.CATHODE 71.91,16.35 71.91,13.97 D1.CATHODE
  Bottom 0.356: v73.34,41.43 71.91,40.01 71.91,18.26 v72.07,18.1
N$21
  Top 0.305: J4.1 62.48,37.85 61.72,38.61 58.67,38.61 58.42,38.86 58.42,40.64 59.44,41.66 67.94,41.66 U$3.1
N$22  (via drill 0.81)
  Top 0.356: v73.18,38.73 68.26,38.73 68.1,38.58 U$3.2
  Bottom 0.356: v73.18,38.73 80.01,31.91 T2.3
N$24  (via drill 0.81)
  Top 0.356: R14.2 81.76,30.48 81.76,26.67 C7.1 81.76,26.51 81.76,23.02 81.28,23.02 T2.2 | v46.04,19.21 46.36,18.89 v61.91,18.89
  Bottom 0.356: v46.04,19.21 46.04,37.47 R15.2 | v61.91,18.89 66.99,13.81 66.99,6.67 69.06,4.6 81.28,4.6 T2.2
N$25  (via drill 0.81)
  Top 0.356: R16.2 45.4,39.69 v45.24,39.69
  Bottom 0.356: v45.24,39.69 44.77,39.21 44.77,17.46 41.91,14.61 R17.1
N$26  (via drill 0.81)
  Top 0.356: v50.96,35.88 37.31,35.88 37.31,34.13 IC1.10
  Bottom 0.356: v50.96,35.88 49.53,37.31 49.53,37.47 R15.1
N$27
  Bottom 0.356: R20.1 14.45,39.37 14.45,43.18 R21.2
N$28  (via drill 0.81)
  Top 0.356: v39.37,14.45 38.89,13.97 37.94,13.97 36.99,13.02 v32.23,13.02
  Bottom 0.356: v39.37,14.45 R17.2 | v32.23,13.02 27.46,8.26 27.46,7.62 J5.3
N$29
  Bottom 0.356: 37.78,45.72 R27.1 | 47.31,45.72 R28.1 48.26,45.72 J8.1
  Bottom 0.406: 37.78,45.72 37.78,49.21 38.1,49.53 39.37,49.53 41.91,52.07 46.99,52.07 48.26,50.8 48.26,45.72
N$30  (via drill 0.81)
  Top 0.356: v20.8,5.4 21.91,4.29 55.25,4.29 57.79,6.83 57.79,7.62 J5.15
  Bottom 0.356: v20.8,5.4 20.8,9.21 21.75,10.16 21.75,13.34 22.38,13.97 R18.1
N$31  (via drill 0.81)
  Top 0.356: 48.1,35.08 39.21,35.08 38.26,34.13 IC1.9 | v57.15,21.75 53.66,21.75 53.34,22.07 53.34,27.94 50.8,30.48 50.8,33.02
  Top 0.406: 48.1,35.08 48.74,35.08 50.8,33.02
  Bottom 0.356: v57.15,21.75 62.07,16.83 62.07,6.03 61.12,5.08 35.08,5.08 35.08,7.62 J5.6
N$32  (via drill 0.81)
  Top 0.356: v68.26,12.38 68.26,13.97 D1.ANODE
  Bottom 0.356: v68.26,12.38 68.26,6.51 69.37,5.4 74.61,5.4 74.61,7.78 J6.2
N$33  (via drill 0.81)
  Top 0.356: v72.87,12.38 70.33,12.38 70.33,14.45 68.26,16.51 D2.ANODE
  Bottom 0.356: v72.87,12.38 77.15,8.1 77.15,7.62 J6.1
N$34
  Bottom 0.356: 11.91,40.96 12.38,40.48 12.38,37.47 14.29,35.56 R19.2
  Bottom 0.406: 11.91,40.96 9.97,40.96 9.65,40.64 9.65,37.08 8.64,37.08 7.62,36.07 R32.1
N$35
  Bottom 0.356: R23.1 R24.2
N$36  (via drill 0.81)
  Top 0.356: v68.42,43.5 70.64,43.5 70.8,43.66 S1.3 | v66.67,28.57 66.52,28.57 66.52,30.64 R13.2
  Bottom 0.356: v68.42,43.5 66.83,41.91 66.83,28.57 | 66.83,28.57 66.83,22.38 Q2.1 | v66.67,28.57 66.83,28.57
N$37
  Top 0.356: R29.2 55.88,37.62 55.88,40.8 R30.2 56.04,40.96 57.15,40.96 J8.3
N$38  (via drill 0.81)
  Top 0.406: R31.1 10.16,7.62 8.64,9.14 8.64,15.75 3.56,20.83 3.56,33.53 4.57,34.54 8.13,34.54 9.14,35.56 9.14,37.08 11.18,39.12 16.76,39.12 v17.27,38.61
  Bottom 0.406: R25.2 v17.27,38.61
N$39
  Bottom 0.356: R31.2 C12.2
N$40
  Top 0.305: U2.D-1 86.98,43.55 SJ1.1
N$42
  Top 0.305: SJ2.1 88.65,45.97 88.9,45.72 88.9,44.45 89.15,44.2 U2.D+1
N$43
  Top 0.406: SJ2.2 85.09,46.48 85.09,48.77 85.34,49.02 87.88,49.02 R33.2
N$45  (via drill 0.81)
  Top 0.356: v62.45,40.16 74.3,40.16 | R34.2 R22.1
  Top 0.406: 74.3,40.16 75.47,40.16 78.49,43.18 85.09,43.18 SJ1.2
  Bottom 0.305: 55.88,35.88 55.88,40.13 56.39,40.64 61.98,40.64 v62.45,40.16
  Bottom 0.356: R34.2 55.88,35.88
PD4  (via drill 0.81)
  Top 0.356: 7.06,26.59 8.57,28.1 R26.3 | 7.06,26.59 6.19,25.72 R26.2 | v14.13,25.4 13.02,26.51 7.14,26.51 7.06,26.59 | v50.96,27.3 47.47,27.3 46.99,27.78 39.69,27.78 IC1.2 | v41.12,11.91 39.37,10.16 31.91,10.16 | 31.91,10.16 30,8.26 30,7.62 J5.4 | v16.99,10.95 17.78,10.16 31.91,10.16
  Bottom 0.356: 16.99,20.8 19.05,20.8 R23.2 | 16.99,20.8 15.24,20.8 C12.1 15.24,20.95 14.13,22.07 v14.13,25.4 | v50.96,27.3 49.85,26.19 49.85,20.64 v41.12,11.91 | v16.99,10.95 16.99,20.8
RESET  (via drill 0.81)
  Top 0.356: v47.31,22.23 35.72,22.23 35.72,25.4 IC1.29 | v48.74,43.97 48.1,44.61 30.8,44.61 28.73,42.55 27.15,42.55 26.67,43.02 26.67,46.35 24.61,46.35 22.86,44.61 U$1.5 v22.86,42.07 | v7.46,21.91 9.05,21.91 9.52,22.38 25.4,22.38 27.15,20.64 S2.1
  Bottom 0.356: v47.31,22.23 49.05,23.97 49.05,35.56 48.1,36.51 48.1,43.34 v48.74,43.97 | R10.1 22.86,37.62 v22.86,42.07 22.86,42.23 23.97,43.34 23.97,51.75 9.84,51.75 4.92,46.83 4.92,24.45 v7.46,21.91
SER  (via drill 0.81)
  Top 0.356: v30.96,22.07 32.39,23.5 33.34,23.5 33.34,25.4 IC1.26 | v34.77,18.26 32.23,15.72 26.19,15.72 23.97,13.49 23.97,12.22 15.72,12.22 | 15.72,12.22 14.92,12.22 10,17.14 v10,19.84 | 91.28,28.1 J9.5 | 75.72,3.49 20.8,3.49 16.51,7.78 16.51,9.68 16.35,9.68 15.72,10.32 15.72,12.22
  Top 0.406: 75.72,3.49 77.15,3.49 88.9,15.24 91.44,15.24 92.96,16.76 92.96,27.43 92.3,28.1 91.28,28.1
  Bottom 0.356: v34.77,18.26 v30.96,22.07 | v10,19.84 10,30.8 10.95,31.75 C11.1 11.11,31.91 11.11,35.56 R19.1 11.11,35.72 11.11,39.37 R20.2
ZVOLT
  Top 0.356: 8.25,40.64 R32.2
  Top 0.406: 8.25,40.64 8.25,43.81 7.62,44.45 7.62,46.99 8.89,48.26 J7.1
